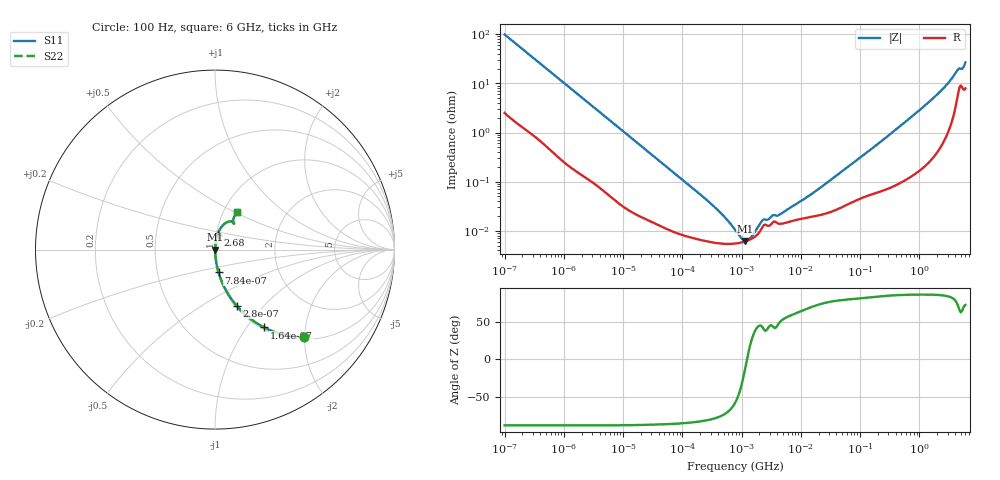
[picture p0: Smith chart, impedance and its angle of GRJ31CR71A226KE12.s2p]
!Murata Part Number: GRJ31CR71A226KE12
!These Parameters are Measured in Series Mode Connection
!Data Generated on Jun 19, 2026
!  o--ll--o
!Port1  Port2
!  o------o
!Operation Temp=25[degC], DC Bias Voltage=0[V]
!Freq. Start=100[Hz] Stop=6[GHz] 401[Steps]
# Hz S RI R 50
!Freq.(Hz) S11(Real) S11(Imag) S21(Real) S21(Imag) S12(Real) S12(Imag) S22(Real) S22(Imag)
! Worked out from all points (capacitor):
!   401 points, 100 Hz to 6 GHz, reference 50 ohm
!   read as one part in series: C = 16.1 uF near 109 Hz
!   lowest |Z| = 6.22 mohm at 1.159 MHz (marker M1)
!   series resonance near 1.235 MHz, so ESL is about 1 nH
!   S11 on the Smith chart (normalised r, x): 100 Hz: 1.05, -1.97; 164 Hz: 1.03, -1.21; 280 Hz: 1.02, -0.72; 784 Hz: 1.01, -0.26; 2.68 GHz: 1.01, +0.17; 6 GHz: 1.16, +0.51
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100  0.4938 -0.4874  0.5062 0.4874  0.5062 0.4874  0.4938 -0.4874
164  0.2744 -0.4339  0.7256 0.4339  0.7256 0.4339  0.2744 -0.4339
280  0.1199 -0.3119  0.8801 0.3119  0.8801 0.3119  0.1199 -0.3119
784  0.0197 -0.1271  0.9803 0.1271  0.9803 0.1271  0.0197 -0.1271
2008  0.00399 -0.0512  0.996 0.0512  0.996 0.0512  0.00399 -0.0512
40335  0.000137 -0.00269  0.9999 0.00269  0.9999 0.00269  0.000137 -0.00269
316350  5.85e-05 -0.000336  0.9999 0.000336  0.9999 0.000336  5.85e-05 -0.000336
495019  5.46e-05 -0.000194  0.9999 0.000194  0.9999 0.000194  5.46e-05 -0.000194
774597  5.51e-05 -9e-05  0.9999 9e-05  0.9999 9e-05  5.51e-05 -9e-05
885955  5.64e-05 -6.3e-05  0.9999 6.3e-05  0.9999 6.3e-05  5.64e-05 -6.3e-05
1159002  6.1e-05 -1.19e-05  0.9999 1.19e-05  0.9999 1.19e-05  6.1e-05 -1.19e-05
1658239  7.51e-05 5.6e-05  0.9999 -5.6e-05  0.9999 -5.6e-05  7.51e-05 5.6e-05
2268635  0.000121 0.000112  0.9999 -0.000112  0.9999 -0.000112  0.000121 0.000112
3394479  0.00015 0.000144  0.9998 -0.000144  0.9998 -0.000144  0.00015 0.000144
4440638  0.000139 0.000165  0.9999 -0.000165  0.9999 -0.000165  0.000139 0.000165
1.555665e7  0.000193 0.000539  0.9998 -0.000539  0.9998 -0.000539  0.000193 0.000539
3.124326e8  0.000818 0.00895  0.9992 -0.00895  0.9992 -0.00895  0.000818 0.00895
1.251881e9  0.00333 0.0354  0.9967 -0.0354  0.9967 -0.0354  0.00333 0.0354
2.679998e9  0.0139 0.0824  0.9861 -0.0824  0.9861 -0.0824  0.0139 0.0824
4.385646e9  0.0746 0.1557  0.9254 -0.1557  0.9254 -0.1557  0.0746 0.1557
5.245841e9  0.1019 0.1467  0.8981 -0.1467  0.8981 -0.1467  0.1019 0.1467
6e9  0.1222 0.2071  0.8778 -0.2071  0.8778 -0.2071  0.1222 0.2071
